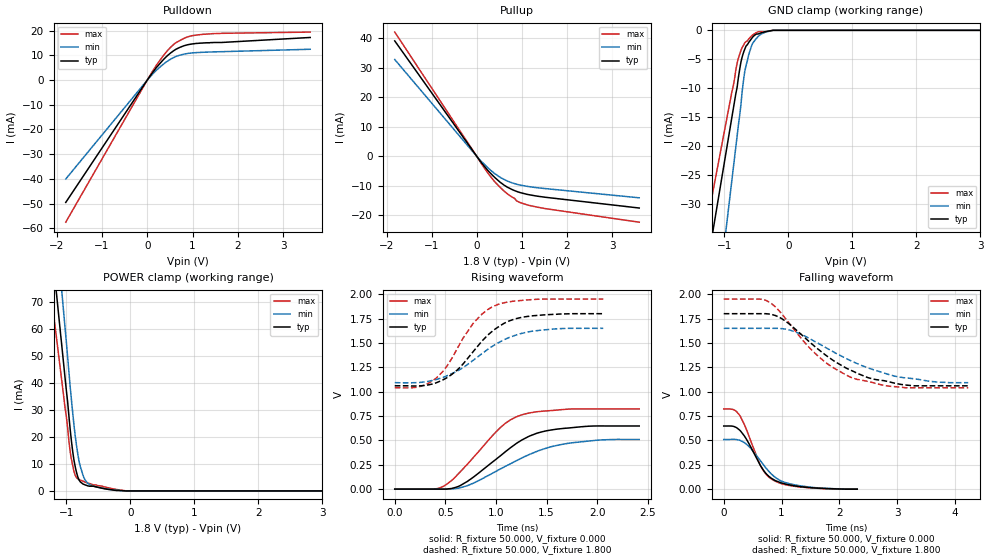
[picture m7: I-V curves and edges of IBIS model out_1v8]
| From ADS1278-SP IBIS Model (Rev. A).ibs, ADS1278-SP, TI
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[Model]   out_1v8
Model_type Output
Vref=0.000E+00
Rref=1.000E+06
Cref=2.000E-11
Vmeas=9.000E-01
C_comp   853.00E-15   853.00E-15   853.00E-15
[Voltage Range]   1.800E+00   1.650E+00   1.950E+00
[POWER Clamp Reference]   1.800E+00   1.650E+00   1.950E+00
[GND Clamp Reference]   0.000E+00   0.000E+00   0.000E+00
[Pullup Reference]   1.800E+00   1.650E+00   1.950E+00
[Pulldown Reference]   0.000E+00   0.000E+00   0.000E+00
[Temperature Range]   25   105   -40
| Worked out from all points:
|   slope of the pulldown table from 0 to 0.27 V, typ, clamps not added: 41.4 ohm
|   slope of the pullup table from 0 to 0.27 V, typ, clamps not added: 52.1 ohm
|   GND clamp passes 1 mA (typ) near -0.54 V on its own axis
|   POWER clamp passes 1 mA (typ) near -0.44 V on its own axis
|   rising waveform, R_fixture 50.000, V_fixture 0.000: 20-80 % time 496ps typ, 603ps min, 438ps max; typ from 0 V to 0.648 V
|   falling waveform, R_fixture 50.000, V_fixture 0.000: 20-80 % time 398ps typ, 454ps min, 356ps max; typ from 0.648 V to 0 V
|   rising waveform, R_fixture 50.000, V_fixture 1.800: 20-80 % time 405ps typ, 490ps min, 349ps max; typ from 1.06 V to 1.8 V
|   falling waveform, R_fixture 50.000, V_fixture 1.800: 20-80 % time 1.02ns typ, 1.2ns min, 922ps max; typ from 1.8 V to 1.06 V
[GND Clamp]
-1.8V     -76.03mA   -112mA     -64.32mA
-1.76V    -73.37mA   -107.9mA   -61.74mA
-880mV    -14.92mA   -25.74mA   -10.53mA
-780mV    -8.152mA   -16.35mA   -4.811mA
-740mV    -5.464mA   -12.8mA    -3.471mA
-720mV    -4.554mA   -10.46mA   -2.931mA
-680mV    -3.236mA   -7.067mA   -2.148mA
-580mV    -1.509mA   -2.848mA   -1.024mA
-500mV    -642uA     -1.411mA   -377.4uA
-420mV    -414.8uA   -620uA     -223.8uA
-240mV    0A         0A         0A
3.6V      0A         0A         0A
[Power Clamp]
-1.82V    228.1mA    268.6mA    180.9mA
-1.76V    214.2mA    258.4mA    173.8mA
-1.04V    46.59mA    65.72mA    34.78mA
-980mV    33.09mA    49.76mA    23.55mA
-940mV    22.81mA    38.69mA    14.52mA
-880mV    11.32mA    24.25mA    7.109mA
-840mV    6.76mA     16.62mA    4.915mA
-800mV    4.02mA     10.77mA    4.178mA
-740mV    2.561mA    5.829mA    3.635mA
-620mV    1.751mA    2.159mA    2.598mA
-180mV    172uA      159uA      390.7uA
3.6V      0A         0A         0A
[Pullup]
-1.82V    39.14mA    32.84mA    42.12mA
100mV     -2.068mA   -1.726mA   -2.419mA
260mV     -5.034mA   -4.057mA   -5.932mA
400mV     -7.161mA   -5.844mA   -8.638mA
520mV     -8.767mA   -7.1mA     -10.52mA
680mV     -10.44mA   -8.348mA   -12.69mA
840mV     -11.6mA    -9.236mA   -14.25mA
880mV     -11.83mA   -9.406mA   -15.04mA
960mV     -12.24mA   -9.701mA   -15.63mA
1.28V     -13.3mA    -10.49mA   -16.98mA
3.6V      -17.47mA   -14.01mA   -22.27mA
[Pulldown]
-1.8V     -49.56mA   -40.07mA   -57.57mA
120mV     3.123mA    2.467mA    3.691mA
360mV     8.369mA    6.513mA    10.02mA
460mV     10.15mA    7.848mA    12.23mA
620mV     12.35mA    9.458mA    15.04mA
900mV     14.36mA    10.83mA    17.59mA
1.24V     15.07mA    11.3mA     18.6mA
3.6V      17.29mA    12.51mA    19.47mA
[Rising Waveform]
R_fixture = 50.000
V_fixture = 0.000
V_fixture_min = 0.000
V_fixture_max = 0.000
|  time   V(typ)   V(min)   V(max)
0s        0V         0V         0V
390ps     0V         0V         842.1uV
490ps     -99.53uV   -298.9uV   34.27mV
595ps     15.65mV    4.881mV    120.8mV
715ps     77.56mV    34.27mV    252.3mV
1.04ns    338.5mV    204.8mV    628.1mV
1.255ns   503.5mV    319.4mV    762.4mV
1.455ns   587.8mV    406.1mV    799.1mV
1.72ns    627.3mV    470.9mV    821.1mV
2.415ns   647.7mV    509.5mV    822.4mV
[Falling Waveform]
R_fixture = 50.000
V_fixture = 0.000
V_fixture_min = 0.000
V_fixture_max = 0.000
|  time   V(typ)   V(min)   V(max)
0s        647.7mV    509.5mV    822.4mV
170ps     643.9mV    510.2mV    815mV
270ps     608.3mV    502.6mV    762.2mV
420ps     484.7mV    447mV      570.7mV
640ps     237.6mV    287mV      236.2mV
730ps     161.4mV    217.4mV    154.6mV
835ps     107.5mV    149.4mV    99.75mV
1.02ns    59.92mV    77.25mV    52.25mV
1.33ns    25.36mV    33.31mV    21.55mV
2.31ns    0V         0V         0V
[Rising Waveform]
R_fixture = 50.000
V_fixture = 1.800
V_fixture_min = 1.650
V_fixture_max = 1.950
|  time   V(typ)   V(min)   V(max)
0s        1.06V      1.092V     1.04V
250ps     1.06V      1.095V     1.053V
405ps     1.089V     1.123V     1.135V
500ps     1.134V     1.156V     1.24V
615ps     1.22V      1.21V      1.438V
780ps     1.417V     1.325V     1.708V
990ps     1.641V     1.482V     1.882V
1.12ns    1.721V     1.551V     1.921V
1.305ns   1.771V     1.61V      1.941V
2.06ns    1.8V       1.65V      1.95V
[Falling Waveform]
R_fixture = 50.000
V_fixture = 1.800
V_fixture_min = 1.650
V_fixture_max = 1.950
|  time   V(typ)   V(min)   V(max)
0s        1.8V       1.65V      1.95V
635ps     1.8V       1.65V      1.949V
790ps     1.796V     1.65V      1.918V
1.075ns   1.721V     1.641V     1.745V
1.62ns    1.442V     1.501V     1.371V
1.905ns   1.316V     1.406V     1.242V
2.235ns   1.21V      1.307V     1.139V
2.505ns   1.142V     1.242V     1.104V
3.17ns    1.066V     1.14V      1.04V
4.23ns    1.06V      1.092V     1.04V
[Ramp]
dV/dt_r   3.904E-01/4.952E-10   3.069E-01/6.026E-10   4.922E-01/4.368E-10
dV/dt_f   4.443E-01/1.025E-09   3.349E-01/1.203E-09   5.460E-01/9.201E-10
R_load = 50
